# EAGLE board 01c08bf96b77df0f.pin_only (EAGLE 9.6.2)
REV: C

Size 25.4 x 17.78 mm. Coordinates in mm from the lower left corner, seen from the top.
Outline: 0,15.24 0,2.54 arc90 2.54,0 22.86,0 arc90 25.4,2.54 25.4,15.24 arc90 22.86,17.78 19.18,17.78 17.4,16 8,16 6.22,17.78 2.54,17.78 arc90 0,15.24
Copper layers (1*16): Top 0.035mm / dielectric 1.5mm / Bottom 0.035mm
Design rules "adafruit *": minimum track width 8mil, minimum drill 15.5mil, track to track 8mil, track to pad 8mil, pad to pad 8mil, via to via 8mil, smd to smd 8mil, copper to edge 10mil, drill to drill 8mil, minimum pad ring 10mil, minimum via ring 8mil, stop-mask expansion 2mil, vias tented up to drill 20mil, thermal gap 10mil
Net classes: 1 highpower: width 0.305 mm, drill 0.483 mm; 2 lowpower: width 0.254 mm, drill 0.483 mm

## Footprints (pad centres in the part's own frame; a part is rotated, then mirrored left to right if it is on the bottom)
CR1220 = smd 3.2 x 3.2: +$1 -8.225,0; +$2 8.225,0 | smd 6.35 x 6.35: - 0,0
0805-NO = smd 1.24 x 1.5: 1 -0.95,0; 2 0.95,0
0603-NO = smd 1.075 x 1: 1 -0.85,0; 2 0.85,0
JST_SH4 = smd 0.6 x 1.55: 1 -1.5,2.514; 2 -0.5,2.514; 3 0.5,2.514; 4 1.5,2.514 | smd 1.2 x 1.8: MT1 -2.8,-1.386; MT2 2.8,-1.386
CHIPLED_0603_NOOUTLINE = smd 0.8 x 0.8: A 0,-0.75; C 0,0.75
FIDUCIAL_1MM = smd 1 x 1: 1 0,0
SO16W = smd 0.6 x 2.2: 1 -4.445,-4.6; 2 -3.175,-4.6; 3 -1.905,-4.6; 4 -0.635,-4.6; 5 0.635,-4.6; 6 1.905,-4.6; 7 3.175,-4.6; 8 4.445,-4.6; 9 4.445,4.6; 10 3.175,4.6; 11 1.905,4.6; 12 0.635,4.6; 13 -0.635,4.6; 14 -1.905,4.6; 15 -3.175,4.6; 16 -4.445,4.6
1X08_ROUND_70 = drill 1 pad 1.778: 1 -8.89,0; 2 -6.35,0; 3 -3.81,0; 4 -1.27,0; 5 1.27,0; 6 3.81,0; 7 6.35,0; 8 8.89,0
SOLDERJUMPER_CLOSEDWIRE = smd 1.168 x 1.6: 1 -0.762,0; 2 0.762,0 | smd 0.635 x 0.203: WIRE 0,0
MOUNTINGHOLE_3.0_PLATEDTHIN = drill 3 pad 3.6: P$1 0,0

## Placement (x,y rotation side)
B1  CR1220  [CR1220]  12.7,10.79 0 bottom
C3  10uF  [0805-NO]  20.07,5.08 0 top
C5  0.1uF  [0603-NO]  1.27,3.68 90 top
CONN3  STEMMA_I2C_QT  [JST_SH4]  22.86,8.89 90 top
CONN4  STEMMA_I2C_QT  [JST_SH4]  2.54,8.89 270 top
D1  GREEN  [CHIPLED_0603_NOOUTLINE]  3.68,12.45 90 top
FID1  FIDUCIAL_1MM  [FIDUCIAL_1MM]  5.08,16.89 0 bottom
FID2  FIDUCIAL_1MM  [FIDUCIAL_1MM]  20.19,1.02 0 bottom
FID3  FIDUCIAL_1MM  [FIDUCIAL_1MM]  20,16.95 0 top
FID4  FIDUCIAL_1MM  [FIDUCIAL_1MM]  1.91,1.14 0 top
IC2  DS3231/SO  [SO16W]  12.38,10.29 90 top
JP1  [1X08_ROUND_70]  12.7,2.54 0 top
R1  10k  [0603-NO]  5.91,5.33 270 top
R2  10k  [0603-NO]  3.68,5.08 180 top
R3  10k  [0603-NO]  5.59,13.46 90 top
SJ1  [SOLDERJUMPER_CLOSEDWIRE]  3.87,5.33 90 bottom
U$1  [ADAFRUIT_2.5MM]  4.64,15.11 0 top
U$9  MOUNTINGHOLE3.0THIN  [MOUNTINGHOLE_3.0_PLATEDTHIN]  2.54,15.24 0 top
U$17  MOUNTINGHOLE3.0THIN  [MOUNTINGHOLE_3.0_PLATEDTHIN]  22.86,15.24 0 top
U$25  [PCBFEAT-REV-040]  1.52,2.54 180 bottom
U$31  [STEMMAQT]  2.92,13.34 270 bottom

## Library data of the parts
B1 C3 C5 CONN3 CONN4 D1 JP1 R1-R3 SJ1 U$1 U$25 = microbuilder
FID1-FID4 = microbuilder; BOM: EXCLUDE
IC2 = adafruit_sensor
U$9 U$17 = adafruit_electromech; BOM: EXCLUDE
U$31 = silks

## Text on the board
tPlace: on | DS3231 RTC | VIN | SCL | VBAT | RST | GND | SDA | 32k | SQW
bPlace: CR1220 3V | VLogic/Vcc: 3-5VDC

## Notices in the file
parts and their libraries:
microbuilder: This work is placed in the public domain, and may be freely used for commercial and non-commercial work with the following conditions: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
